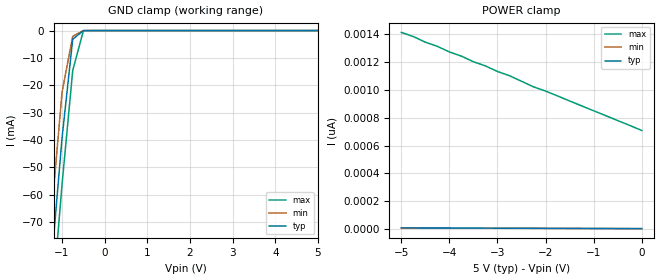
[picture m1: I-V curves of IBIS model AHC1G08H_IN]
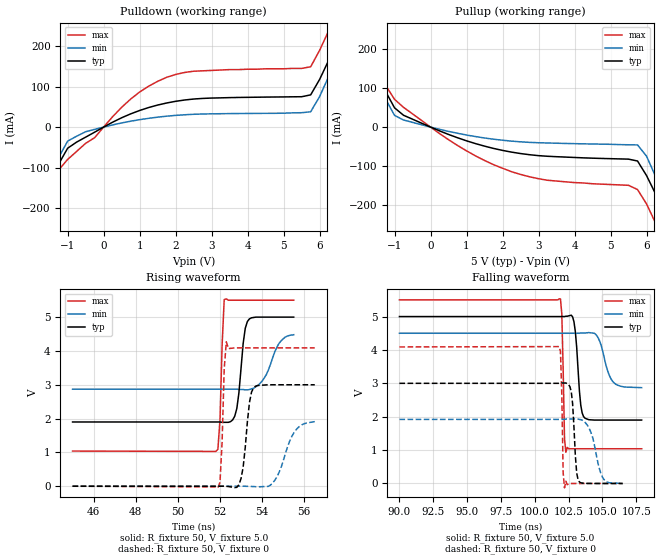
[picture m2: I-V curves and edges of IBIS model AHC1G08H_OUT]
| TEXAS INSTRUMENTS INCORPORATED
| Standard Linear and Logic Group
| IBIS Model of SN74AHC1G08H
| SINGLE 2-INPUT POSITIVE-AND GATE
| MPAK-5 5-pin (DBV) Package
[IBIS Ver]   2.1
[Comment Char]  |_char
[File name]   ul08_5m.ibs
[File Rev]   2.0
[Date]   April 17, 2000
[Source]   Data created from SPICE simulations at Hitachi,Ltd.
[Notes]   The following is an IBIS List for the AHC1G08H.
|   Please contact sllibis@ti.com with questions and
|   comments concerning SLL IBIS models.
[Disclaimer] Property of Texas Instruments Incorporated.  Unauthorized
   reproduction and/or distribution is strictly prohibited.
   This product is protected under copyright law.
   Created 2000, (C) Copyright 2000, Texas Instruments Inc.,
   All Rights Reserved.
   UNLESS THERE IS A SIGNED, WRITTEN AGREEMENT TO THE
   CONTRARY, TEXAS INSTRUMENTS () IS PROVIDING THE IBIS
   MODELS  AND WITHOUT ANY WARRANTY, EXPRESSED OR
   IMPLIED.  TI assumes no liability for:
   1) the accuracy of the IBIS models provided to your
   company;
   2) the proper functioning of these IBIS Models in your
   design or for any resulting applications; or
   3) infringement of patents, copyrights or intellectual
   property rights resulting from your use of these IBIS
   models.
   TI provides IBIS Models as a service to our customers.
   You and your company shall not distribute, sell or give
   these models to anyone else without prior written
   permission from TI.
   TI reserves the right to make changes to our products or
   to discontinue any semiconductor product or service
   without notice, and advises our customers to obtain the
   latest version of relevant information to verify, before
   placing orders, that the information being relied on is
   current.
   Please be aware that your receipt and use of the IBIS
   information provided shall serve as acceptance of these
   terms and conditions.  If you do not accept these terms,
   you should return or destroy the IBIS models and any
   other accompanying information immediately.
|   Component AHC1G08H
[Component]   AHC1G08H
[Manufacturer]   Hitachi, Ltd.
[Package]
|   typ   min   max
R_pkg   0.089   0.050   0.104
L_pkg   1.520nH   0.920nH   1.720nH
C_pkg   0.240pF   0.150pF   0.520pF
[Pin]   signal_name   model_name   R_pin   L_pin   C_pin
1   A   AHC1G08H_IN   0.097   1.620nH   0.150pF
2   B   AHC1G08H_IN   0.050   0.920nH   0.210pF
3   GND   GND   0.092   1.640nH   0.520pF
4   Y   AHC1G08H_OUT   0.104   1.720nH   0.160pF
5   VCC   POWER   0.103   1.710nH   0.150pF
| Models and submodels in the file (2): AHC1G08H_IN (Input), AHC1G08H_OUT (Output)
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|   Model AHC1G08H_IN
[Model]   AHC1G08H_IN
Model_type  Input
Polarity   Inverting
Vinl = 1.50
Vinh = 3.50
| variable   typ   min   max
C_comp   2.19pF   2.07pF   2.30pF
[Temperature Range]   25   85   -40
[Voltage Range]   5.0   4.5   5.5
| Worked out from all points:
|   GND clamp passes 1 mA (typ) near -0.58 V on its own axis
[GND Clamp]
|   Voltage   I(typ)   I(min)   I(max)
-5V       -823mA     -807mA     -840mA
-1.5V     -133mA     -115mA     -150mA
-1.25V    -85.2mA    -67.5mA    -103mA
-1V       -39.2mA    -22.5mA    -56.2mA
-750mV    -3.18mA    -2.09mA    -14.6mA
-500mV    -11.6uA    -2.99uA    -57.1uA
5V        5.34pA     5pA        708pA
[POWER Clamp]
|   Voltage   I(typ)   I(min)   I(max)
-5V       10.6pA     10pA       1.41nA
-4.75V    10.3pA     9.75pA     1.38nA
-4.5V     10pA       9.5pA      1.34nA
-4.25V    9.78pA     9.25pA     1.31nA
-4V       9.52pA     9pA        1.27nA
-3.75V    9.26pA     8.75pA     1.24nA
-3.5V     9pA        8.5pA      1.2nA
-3.25V    8.74pA     8.25pA     1.17nA
-2.75V    8.21pA     7.75pA     1.1nA
-2.25V    7.69pA     7.25pA     1.02nA
-2V       7.43pA     7pA        990pA
0V        5.34pA     5pA        708pA
|   Model AHC1G08H_OUT
[Model]   AHC1G08H_OUT
Model_type  Output
Polarity   Inverting
Vmeas = 2.5
Cref = 15pf
| variable   typ   min   max
C_comp   4.52pF   4.32pF   4.72pF
[Temperature Range]   25   85   -40
[Voltage Range]   5.0   4.5   5.5
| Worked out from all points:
|   slope of the pulldown table from 0 to 0.75 V, typ, clamps not added: 23 ohm
|   slope of the pullup table from 0 to 0.75 V, typ, clamps not added: 27.3 ohm
|   rising waveform, R_fixture 50, V_fixture 5.0: 20-80 % time 289ps typ, 653ps min, 136ps max; typ from 1.9 V to 5 V
|   falling waveform, R_fixture 50, V_fixture 5.0: 20-80 % time 324ps typ, 682ps min, 143ps max; typ from 5 V to 1.9 V
|   falling waveform, R_fixture 50, V_fixture 0: 20-80 % time 251ps typ, 677ps min, 126ps max; typ from 3 V to 0 V
|   rising waveform, R_fixture 50, V_fixture 0: 20-80 % time 281ps typ, 677ps min, 132ps max; typ from 0 V to 3 V
[Pulldown]
|   Voltage   I(typ)   I(min)   I(max)
-5V       -826mA     -810mA     -842mA
-2.25V    -282mA     -267mA     -299mA
-2V       -234mA     -219mA     -250mA
-1.25V    -91.3mA    -75.2mA    -106mA
-1V       -52.3mA    -34.7mA    -80mA
750mV     32.6mA     14.5mA     69.2mA
1.75V     59.5mA     26.9mA     123mA
5.75V     79.6mA     37.8mA     149mA
6.25V     165mA      125mA      238mA
6.75V     261mA      217mA      336mA
7V        310mA      265mA      385mA
10V       906mA      861mA      980mA
[Pullup]
|   Voltage   I(typ)   I(min)   I(max)
-5V       828mA      811mA      845mA
-2.25V    284mA      267mA      301mA
-2V       235mA      218mA      252mA
-1V       49.6mA     30.1mA     71.4mA
750mV     -27.5mA    -16mA      -47.4mA
2.25V     -64.5mA    -36.2mA    -115mA
5.75V     -87.4mA    -46mA      -161mA
6V        -125mA     -75mA      -198mA
6.25V     -172mA     -127mA     -247mA
6.75V     -269mA     -224mA     -345mA
7V        -318mA     -273mA     -395mA
10V       -917mA     -874mA     -991mA
[Ramp]
| variable   typ   min   max
dV/dt_r   1.80E+00/2.80E-10   1.15E+00/6.80E-10   2.45E+00/1.30E-10
dV/dt_f   1.86E+00/3.20E-10   9.76E-01/6.70E-10   2.68E+00/1.40E-10
R_load = 50
[Rising Waveform]
R_fixture = 50
V_fixture = 5.0
V_fixture_min = 4.5
V_fixture_max = 5.5
|   Time   V(typ)   V(min)   V(max)
45ns      1.9V       2.87V      1.04V
51.8ns    1.9V       2.87V      1.03V
51.9ns    1.9V       2.87V      1.09V
52ns      1.9V       2.87V      1.96V
52.1ns    1.89V      2.87V      4.16V
52.2ns    1.89V      2.87V      5.52V
52.8ns    2.3V       2.87V      5.5V
53.1ns    4.22V      2.86V      5.5V
53.3ns    4.87V      2.85V      5.5V
55.5ns    5V         4.48V      5.5V
[Falling Waveform]
R_fixture = 50
V_fixture = 5.0
V_fixture_min = 4.5
V_fixture_max = 5.5
|   Time   V(typ)   V(min)   V(max)
90ns      5V         4.5V       5.5V
101.9ns   5V         4.5V       5.53V
102ns     5V         4.5V       5.08V
102.2ns   5V         4.5V       1.34V
102.3ns   5.01V      4.5V       934mV
102.9ns   4.84V      4.5V       1.04V
103.6ns   2.01V      4.51V      1.04V
104.6ns   1.9V       4.42V      1.04V
105.9ns   1.9V       3V         1.04V
107.9ns   1.9V       2.87V      1.04V
[Falling Waveform]
R_fixture = 50
V_fixture = 0
|   Time   V(typ)   V(min)   V(max)
90ns      3V         1.92V      4.09V
101.8ns   3V         1.92V      4.1V
101.9ns   3V         1.92V      3.96V
102ns     3.01V      1.92V      2.66V
102.1ns   3.01V      1.92V      322mV
102.2ns   3.01V      1.92V      -131mV
102.7ns   2.75V      1.93V      -158uV
103.2ns   114mV      1.93V      125uV
105.1ns   311uV      127mV      -96uV
106.5ns   130uV      1.43mV     -63uV
[Rising Waveform]
R_fixture = 50
V_fixture = 0
|   Time   V(typ)   V(min)   V(max)
45ns      0V         0V         0V
51.9ns    285uV      -17uV      -47.7mV
52ns      826uV      -20uV      120mV
52.1ns    1.27mV     -22uV      1.3V
52.2ns    1.15mV     -30uV      3.47V
52.3ns    -1.8mV     -6uV       4.27V
53ns      230mV      1.16mV     4.09V
53.6ns    2.91V      -10.7mV    4.09V
54.5ns    3V         95.3mV     4.09V
56.5ns    3V         1.91V      4.09V
